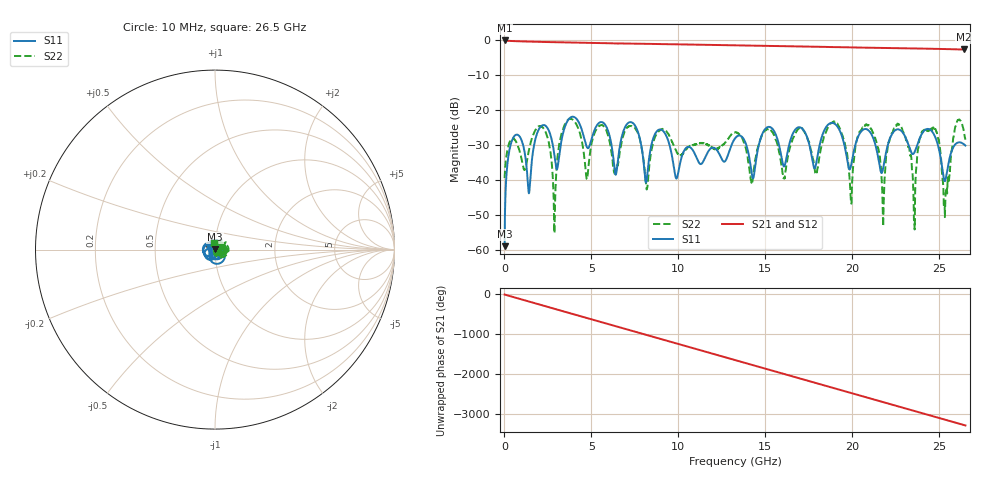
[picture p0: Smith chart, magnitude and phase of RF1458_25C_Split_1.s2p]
!Keysight Technologies,N5245B,MY55451909,A.13.80.08
!Automatic Fixture Removal (AFR)
!Date: Thursday, August 27, 2020, 03:54:42
!S2P File: Measurements: S11,S21,S12,S22:
# MHz S  RI  R 50
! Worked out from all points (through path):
!   2650 points, 10 MHz to 26.5 GHz, reference 50 ohm
!   highest |S21| = -0.01 dB at 10 MHz (marker M1); lowest = -2.6 dB at 26.41 GHz (marker M2)
!   group delay of S21, straight-line fit = 343 ps
!   lowest |S11| = -58.9 dB at 10 MHz (marker M3), VSWR 1.00, Z = 50 + j0.112 ohm
!   |S11| at or under -10 dB: start of sweep to end of sweep
!   |S22| runs from -55.2 to -22.4 dB; largest |S21 - S12| = 1.5e-15
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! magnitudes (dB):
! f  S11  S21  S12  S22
! 10 MHz  -58.9  0.0  0.0  -39.4
! 580 MHz  -27.3  -0.2  -0.2  -28.4
! 1.41 GHz  -43.8  -0.3  -0.3  -31.3
! 2.24 GHz  -24.2  -0.4  -0.4  -25.1
! 2.87 GHz  -32.7  -0.5  -0.5  -55.2
! 3.5 GHz  -24.4  -0.6  -0.6  -23.8
! 4.43 GHz  -25.3  -0.7  -0.7  -28.3
! 7.4 GHz  -23.7  -0.9  -0.9  -24.7
! 8.19 GHz  -39.5  -1.0  -1.0  -42.3
! 8.84 GHz  -25.7  -1.0  -1.0  -26.2
! 13.26 GHz  -28.0  -1.4  -1.4  -26.3
! 17.67 GHz  -33.3  -1.8  -1.8  -32.4
! 19.05 GHz  -24.1  -1.9  -1.9  -23.4
! 19.92 GHz  -36.0  -2.0  -2.0  -46.1
! 20.89 GHz  -25.6  -2.1  -2.1  -24.2
! 21.77 GHz  -36.7  -2.1  -2.1  -53.2
! 22.09 GHz  -29.1  -2.2  -2.2  -29.3
! 23.56 GHz  -32.2  -2.3  -2.3  -51.5
! 24.74 GHz  -27.4  -2.4  -2.4  -25.4
! 25.34 GHz  -40.2  -2.5  -2.5  -46.9
! 26.41 GHz  -29.7  -2.6  -2.6  -26.0
! 26.5 GHz  -30.1  -2.6  -2.6  -28.4
